| IBIS file 71v35761z_pf.ibs created by s2ibis2 version 1.1
| North Carolina State University Electronics Research Laboratory  1995
[IBIS ver]   2.1
[File name]   71v35761z_pf.ibs
[File Rev]   1.1
[Date]   8/15/00
[Source]   Integrated Device Technology, Inc.
[Notes]   1. Temperatures: typ=25C, min=70C, max=0C 2. Cemos10_3v
   process. 3. Ramp rates based on 50 ohm load.
[Copyright]   Copyright 2000, Integrated Device Technology, Inc. Integrated
   Device Technology, Inc. ("IDT") hereby grants the user of this
   IBIS model a non-exclusive, nontransferable license to use
   this IBIS model under the following terms. The user is granted
   this license only to use the IBIS model and is not granted
   rights to sell, copy (except as needed to run the IBIS model),
   rent, lease or sub-license the IBIS model in whole or in part,
   or in modified form to anyone. The User may modify the IBIS
   model to suit its specific applications, but rights to
   derivative works and such modifications shall belong to IDT.
   This IBIS model is provided on an AS IS" basis and IDT makes
   absolutely no warranty with respect to the information
   contained herein. IDT DISCLAIMS AND CUSTOMER WAIVES ALL
   WARRANTIES, EXPRESS AND IMPLIED, INCLUDING WARRANTIES OF
   MERCHANTABILITY AND FITNESS FOR A PARTICULAR PURPOSE. THE
   ENTIRE RISK AS TO QUALITY AND PERFORMANCE IS WITH THE USER
   ACCORDINGLY, IN NO EVENT SHALL IDT BE LIABLE FOR ANY DIRECT OR
   INDIRECT DAMAGES, WHETHER IN CONTRACT OR TORT, INCLUDING ANY
   LOST PROFITS OR OTHER INCIDENTAL, CONSEQUENTIAL, EXEMPLARY, OR
   PUNITIVE DAMAGES ARISING OUT OF THE USE OR APPLICATION OF THE
   IBIS model. Further, IDT reserves the right to make changes
   without notice to any product herein to improve reliability,
   function, or design. IDT does not convey any license under
   patent rights or any other intellectual property rights,
   including those of third parties. IDT is not obligated to
   provide maintenance or support for the licensed IBIS model.
|   Component idt71V35761Z
[Component]   idt71V35761Z
[Manufacturer]   Integrated Device Technology
|   This component uses the 100 pin TQFP package (PF)
[Package]
| variable   typ   min   max
R_pkg   0.000   0.000   0.000
L_pkg   0.000H   0.000H   0.000H
C_pkg   0.000F   0.000F   0.000F
[Pin]  signal_name   model_name   R_pin   L_pin   C_pin
1   IOP3   IOPAD35761Z   6.37e-03  4.62e-09  9.13e-13
2   IO16   IOPAD35761Z   6.36e-03  4.72e-09  1.09e-12
3   IO17   IOPAD35761Z   6.49e-03  4.81e-09  1.14e-12
4   VDDQ   POWER   6.57e-03  4.90e-09  1.20e-12
5   VSS   GND   6.69e-03  4.70e-09  1.16e-12
6   IO18   IOPAD35761Z   6.36e-03  4.36e-09  1.09e-12
7   IO19   IOPAD35761Z   6.06e-03  4.05e-09  1.02e-12
8   IO20   IOPAD35761Z   5.76e-03  3.71e-09  9.52e-13
9   IO21   IOPAD35761Z   5.42e-03  3.37e-09  8.84e-13
10   VSS   GND   5.15e-03  3.07e-09  8.06e-13
11   VDDQ   POWER   4.86e-03  2.78e-09  7.49e-13
12   IO22   IOPAD35761Z   4.57e-03  2.51e-09  6.83e-13
13   IO23   IOPAD35761Z   4.27e-03  2.27e-09  6.18e-13
14   VDD   POWER   4.04e-03  2.09e-09  5.49e-13
15   VDD   POWER   3.63e-03  1.93e-09  3.51e-13
16   NC   NC   3.63e-03  1.93e-09  3.51e-13
17   VSS   GND   4.04e-03  2.09e-09  5.49e-13
18   IO24   IOPAD35761Z   4.27e-03  2.27e-09  6.18e-13
19   IO25   IOPAD35761Z   4.57e-03  2.51e-09  6.83e-13
20   VDDQ   POWER   4.86e-03  2.78e-09  7.49e-13
21   VSS   GND   5.15e-03  3.07e-09  8.06e-13
22   IO26   IOPAD35761Z   5.42e-03  3.37e-09  8.84e-13
23   IO27   IOPAD35761Z   5.76e-03  3.71e-09  9.52e-13
24   IO28   IOPAD35761Z   6.06e-03  4.05e-09  1.02e-12
25   IO29   IOPAD35761Z   6.36e-03  4.36e-09  1.09e-12
26   VSS   GND   6.69e-03  4.70e-09  1.16e-12
27   VDDQ   POWER   6.57e-03  4.90e-09  1.20e-12
28   IO30   IOPAD35761Z   6.49e-03  4.81e-09  1.14e-12
29   IO31   IOPAD35761Z   6.36e-03  4.72e-09  1.09e-12
30   IOP4   IOPAD35761Z   6.37e-03  4.62e-09  9.13e-13
31   NLBO   INPAD_71V35761Z   4.41e-03  4.16e-09  7.09e-13
32   A5   INPAD_71V35761Z   4.39e-03  4.03e-09  7.72e-13
33   A4   INPAD_71V35761Z   4.30e-03  3.88e-09  7.35e-13
34   A3   INPAD_71V35761Z   4.21e-03  3.73e-09  7.18e-13
35   A2   INPAD_71V35761Z   4.13e-03  3.60e-09  7.07e-13
36   A1   INPAD_71V35761Z   4.09e-03  3.51e-09  6.95e-13
37   A0   INPAD_71V35761Z   4.04e-03  3.41e-09  6.83e-13
38   NC   NC   3.99e-03  3.31e-09  6.74e-13
39   NC   NC   3.93e-03  3.23e-09  6.62e-13
40   VSS   GND   3.95e-03  3.18e-09  4.49e-13
41   VDD   POWER   3.95e-03  3.18e-09  4.49e-13
42   NC   NC   3.93e-03  3.23e-09  6.62e-13
43   NC   NC   3.99e-03  3.31e-09  6.74e-13
44   A10   INPAD_71V35761Z   4.04e-03  3.41e-09  6.83e-13
45   A11   INPAD_71V35761Z   4.09e-03  3.51e-09  6.95e-13
46   A12   INPAD_71V35761Z   4.13e-03  3.60e-09  7.07e-13
47   A13   INPAD_71V35761Z   4.21e-03  3.73e-09  7.18e-13
48   A14   INPAD_71V35761Z   4.30e-03  3.88e-09  7.35e-13
49   A15   INPAD_71V35761Z   4.39e-03  4.03e-09  7.72e-13
50   A16   INPAD_71V35761Z   4.41e-03  4.16e-09  7.09e-13
51   IOP1   IOPAD35761Z   6.37e-03  4.62e-09  9.13e-13
52   IO0   IOPAD35761Z   6.36e-03  4.72e-09  1.09e-12
53   IO1   IOPAD35761Z   6.49e-03  4.81e-09  1.14e-12
54   VDDQ   POWER   6.57e-03  4.90e-09  1.20e-12
55   VSS   GND   6.69e-03  4.70e-09  1.16e-12
56   IO2   IOPAD35761Z   6.36e-03  4.36e-09  1.09e-12
57   IO3   IOPAD35761Z   6.06e-03  4.05e-09  1.02e-12
58   IO4   IOPAD35761Z   5.76e-03  3.71e-09  9.52e-13
59   IO5   IOPAD35761Z   5.42e-03  3.37e-09  8.84e-13
60   VSS   GND   5.15e-03  3.07e-09  8.06e-13
61   VDDQ   POWER   4.86e-03  2.78e-09  7.49e-13
62   IO6   IOPAD35761Z   4.57e-03  2.51e-09  6.83e-13
63   IO7   IOPAD35761Z   4.27e-03  2.27e-09  6.18e-13
64   ZZ   INPAD_71V35761Z   4.04e-03  2.09e-09  5.49e-13
65   VDD   POWER   3.63e-03  1.93e-09  3.51e-13
66   NC   NC   3.63e-03  1.93e-09  3.51e-13
67   VSS   GND   4.04e-03  2.09e-09  5.49e-13
68   IO8   IOPAD35761Z   4.27e-03  2.27e-09  6.18e-13
69   IO9   IOPAD35761Z   4.57e-03  2.51e-09  6.83e-13
70   VDDQ   POWER   4.86e-03  2.78e-09  7.49e-13
71   VSS   GND   5.15e-03  3.07e-09  8.06e-13
72   IO10   IOPAD35761Z   5.42e-03  3.37e-09  8.84e-13
73   IO11   IOPAD35761Z   5.76e-03  3.71e-09  9.52e-13
74   IO12   IOPAD35761Z   6.06e-03  4.05e-09  1.02e-12
75   IO13   IOPAD35761Z   6.36e-03  4.36e-09  1.09e-12
76   VSS   GND   6.69e-03  4.70e-09  1.16e-12
77   VDDQ   POWER   6.57e-03  4.90e-09  1.20e-12
78   IO14   IOPAD35761Z   6.49e-03  4.81e-09  1.14e-12
79   IO15   IOPAD35761Z   6.36e-03  4.72e-09  1.09e-12
80   IOP2   IOPAD35761Z   6.37e-03  4.62e-09  9.13e-13
81   A9   INPAD_71V35761Z   4.41e-03  4.16e-09  7.09e-13
82   A8   INPAD_71V35761Z   4.39e-03  4.03e-09  7.72e-13
83   NADV   INPAD_71V35761Z   4.30e-03  3.88e-09  7.35e-13
84   NADSP   INPAD_71V35761Z   4.21e-03  3.73e-09  7.18e-13
85   NADSC   INPAD_71V35761Z   4.13e-03  3.60e-09  7.07e-13
86   NOE   INPAD_71V35761Z   4.09e-03  3.51e-09  6.95e-13
87   NBWE   INPAD_71V35761Z   4.04e-03  3.41e-09  6.83e-13
88   NGW   INPAD_71V35761Z   3.99e-03  3.31e-09  6.74e-13
89   CLK   INCLK_71V35761Z   3.93e-03  3.23e-09  6.62e-13
90   VSS   GND   3.95e-03  3.18e-09  4.49e-13
91   VDD   POWER   3.95e-03  3.18e-09  4.49e-13
92   NCS1   INPAD_71V35761Z   3.93e-03  3.23e-09  6.62e-13
93   NBW1   INPAD_71V35761Z   3.99e-03  3.31e-09  6.74e-13
94   NBW2   INPAD_71V35761Z   4.04e-03  3.41e-09  6.83e-13
95   NBW3   INPAD_71V35761Z   4.09e-03  3.51e-09  6.95e-13
96   NBW4   INPAD_71V35761Z   4.13e-03  3.60e-09  7.07e-13
97   CS0   INPAD_71V35761Z   4.21e-03  3.73e-09  7.18e-13
98   NCE   INPAD_71V35761Z   4.30e-03  3.88e-09  7.35e-13
99   A7   INPAD_71V35761Z   4.39e-03  4.03e-09  7.72e-13
100   A6   INPAD_71V35761Z   4.41e-03  4.16e-09  7.09e-13
1000   GNDQ   GND
| IOIN IOIN   dummy_model
| OC   OC   dummy_model
| IN   IN   dummy_model
| CLK  CLK   dummy_model
[Pin Mapping]  pulldown_ref   pullup_ref   gnd_clamp_ref   power_clamp_ref
1   EXTGNDQ   EXTVDDQ   EXTGND   EXTVDD
2   EXTGNDQ   EXTVDDQ   EXTGND   EXTVDD
3   EXTGNDQ   EXTVDDQ   EXTGND   EXTVDD
4   NC   EXTVDDQ
5   EXTGND   NC
6   EXTGNDQ   EXTVDDQ   EXTGND   EXTVDD
7   EXTGNDQ   EXTVDDQ   EXTGND   EXTVDD
8   EXTGNDQ   EXTVDDQ   EXTGND   EXTVDD
9   EXTGNDQ   EXTVDDQ   EXTGND   EXTVDD
10   EXTGND   NC
11   NC   EXTVDDQ
12   EXTGNDQ   EXTVDDQ   EXTGND   EXTVDD
13   EXTGNDQ   EXTVDDQ   EXTGND   EXTVDD
14   NC   EXTVDD
15   NC   EXTVDD
16   NC   NC   NC   NC
17   EXTGND   NC
18   EXTGNDQ   EXTVDDQ   EXTGND   EXTVDD
19   EXTGNDQ   EXTVDDQ   EXTGND   EXTVDD
20   NC   EXTVDDQ
21   EXTGND   NC
22   EXTGNDQ   EXTVDDQ   EXTGND   EXTVDD
23   EXTGNDQ   EXTVDDQ   EXTGND   EXTVDD
24   EXTGNDQ   EXTVDDQ   EXTGND   EXTVDD
25   EXTGNDQ   EXTVDDQ   EXTGND   EXTVDD
26   EXTGND   NC
27   NC   EXTVDDQ
28   EXTGNDQ   EXTVDDQ   EXTGND   EXTVDD
29   EXTGNDQ   EXTVDDQ   EXTGND   EXTVDD
30   EXTGNDQ   EXTVDDQ   EXTGND   EXTVDD
31   EXTGNDQ   EXTVDDQ   EXTGND   EXTVDD
32   EXTGNDQ   EXTVDDQ   EXTGND   EXTVDD
33   EXTGNDQ   EXTVDDQ   EXTGND   EXTVDD
34   EXTGNDQ   EXTVDDQ   EXTGND   EXTVDD
35   EXTGNDQ   EXTVDDQ   EXTGND   EXTVDD
36   EXTGNDQ   EXTVDDQ   EXTGND   EXTVDD
37   EXTGNDQ   EXTVDDQ   EXTGND   EXTVDD
38   NC   NC   NC   NC
39   NC   NC   NC   NC
40   EXTGND   NC
41   NC   EXTVDD
42   NC   NC   NC   NC
43   NC   NC   NC   NC
44   EXTGNDQ   EXTVDDQ   EXTGND   EXTVDD
45   EXTGNDQ   EXTVDDQ   EXTGND   EXTVDD
46   EXTGNDQ   EXTVDDQ   EXTGND   EXTVDD
47   EXTGNDQ   EXTVDDQ   EXTGND   EXTVDD
48   EXTGNDQ   EXTVDDQ   EXTGND   EXTVDD
49   EXTGNDQ   EXTVDDQ   EXTGND   EXTVDD
50   EXTGNDQ   EXTVDDQ   EXTGND   EXTVDD
51   EXTGNDQ   EXTVDDQ   EXTGND   EXTVDD
52   EXTGNDQ   EXTVDDQ   EXTGND   EXTVDD
53   EXTGNDQ   EXTVDDQ   EXTGND   EXTVDD
54   NC   EXTVDDQ
55   EXTGND   NC
56   EXTGNDQ   EXTVDDQ   EXTGND   EXTVDD
57   EXTGNDQ   EXTVDDQ   EXTGND   EXTVDD
58   EXTGNDQ   EXTVDDQ   EXTGND   EXTVDD
59   EXTGNDQ   EXTVDDQ   EXTGND   EXTVDD
60   EXTGND   NC
61   NC   EXTVDDQ
62   EXTGNDQ   EXTVDDQ   EXTGND   EXTVDD
63   EXTGNDQ   EXTVDDQ   EXTGND   EXTVDD
64   EXTGNDQ   EXTVDDQ   EXTGND   EXTVDD
65   NC   EXTVDD
66   NC   NC   NC   NC
67   EXTGND   NC
68   EXTGNDQ   EXTVDDQ   EXTGND   EXTVDD
69   EXTGNDQ   EXTVDDQ   EXTGND   EXTVDD
70   NC   EXTVDDQ
71   EXTGND   NC
72   EXTGNDQ   EXTVDDQ   EXTGND   EXTVDD
73   EXTGNDQ   EXTVDDQ   EXTGND   EXTVDD
74   EXTGNDQ   EXTVDDQ   EXTGND   EXTVDD
75   EXTGNDQ   EXTVDDQ   EXTGND   EXTVDD
76   EXTGND   NC
77   NC   EXTVDDQ
78   EXTGNDQ   EXTVDDQ   EXTGND   EXTVDD
79   EXTGNDQ   EXTVDDQ   EXTGND   EXTVDD
80   EXTGNDQ   EXTVDDQ   EXTGND   EXTVDD
81   EXTGNDQ   EXTVDDQ   EXTGND   EXTVDD
82   EXTGNDQ   EXTVDDQ   EXTGND   EXTVDD
83   EXTGNDQ   EXTVDDQ   EXTGND   EXTVDD
84   EXTGNDQ   EXTVDDQ   EXTGND   EXTVDD
85   EXTGNDQ   EXTVDDQ   EXTGND   EXTVDD
86   EXTGNDQ   EXTVDDQ   EXTGND   EXTVDD
87   EXTGNDQ   EXTVDDQ   EXTGND   EXTVDD
88   EXTGNDQ   EXTVDDQ   EXTGND   EXTVDD
89   EXTGNDQ   EXTVDDQ   EXTGND   EXTVDD
90   EXTGND   NC
91   NC   EXTVDD
92   EXTGNDQ   EXTVDDQ   EXTGND   EXTVDD
93   EXTGNDQ   EXTVDDQ   EXTGND   EXTVDD
94   EXTGNDQ   EXTVDDQ   EXTGND   EXTVDD
95   EXTGNDQ   EXTVDDQ   EXTGND   EXTVDD
96   EXTGNDQ   EXTVDDQ   EXTGND   EXTVDD
97   EXTGNDQ   EXTVDDQ   EXTGND   EXTVDD
98   EXTGNDQ   EXTVDDQ   EXTGND   EXTVDD
99   EXTGNDQ   EXTVDDQ   EXTGND   EXTVDD
100   EXTGNDQ   EXTVDDQ   EXTGND   EXTVDD
1000   EXTGNDQ   NC
| Models and submodels in the file (3): IOPAD35761Z (I/O), INCLK_71V35761Z (Input), INPAD_71V35761Z (Input)
